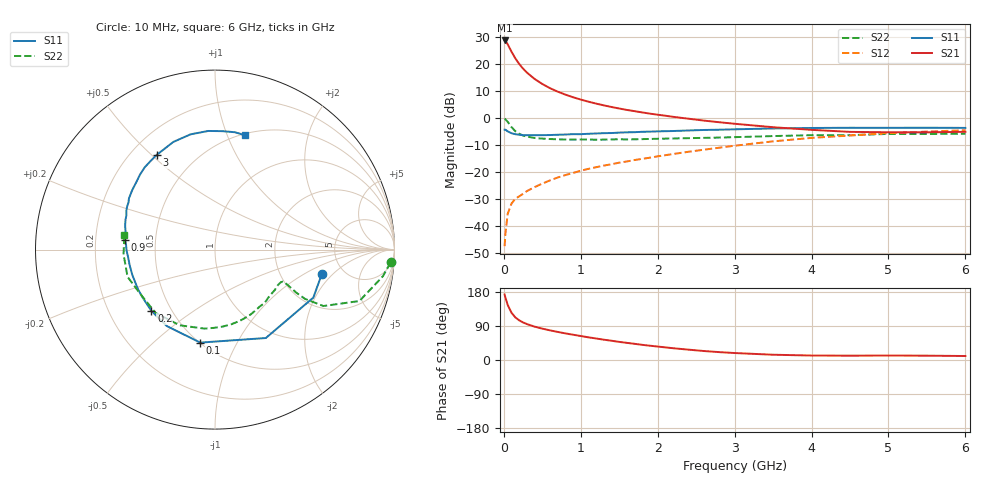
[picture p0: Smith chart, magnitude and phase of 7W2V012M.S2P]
! Infineon Technologies  Discrete & RF Semiconductors
! BFS17W
! Si NPN RF Bipolar Junction Transistor in SOT323
! VCE = 2 V  IC = 12 mA
! Common Emitter S-Parameters:  August  1999
# GHz  S  MA  R  50
!  f  S11  S21  S12  S22
! GHz  MAG  ANG  MAG  ANG  MAG  ANG  MAG  ANG
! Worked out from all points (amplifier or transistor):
!   36 points, 10 MHz to 6 GHz, reference 50 ohm
!   highest |S21| = 28.7 dB at 10 MHz (marker M1)
!   |S21| within 3 dB of that: start of sweep to 78.9 MHz
!   unconditionally stable (mu >= 1): 344.6 MHz to 2.89 GHz; 4.095 GHz to end of sweep
!   at 250 MHz: K = 0.88, MSG = 23.1 dB, |S12| = -28.0 dB
!   at 1.4 GHz: K = 1.24, MAG = 7.6 dB, |S12| = -17.0 dB
!   at 6 GHz: K = 1.09, MAG = -2.1 dB, |S12| = -4.5 dB
!   S11 on the Smith chart (normalised r, x): 10 MHz: 3.43, -1.50; 100 MHz: 0.50, -0.72; 200 MHz: 0.39, -0.35; 900 MHz: 0.33, +0.05; 3 GHz: 0.30, +0.52; 6 GHz: 0.51, +1.16
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0.01  0.6103 -13.0  27.17 172.8  0.0043 84.0  0.9805 -4.2
0.02  0.6098 -26.0  26.55 164.9  0.0072 81.8  0.9475 -9.0
0.05  0.5682 -60.1  23.09 145.4  0.017 67.1  0.8541 -19.6
0.1  0.5247 -99.0  16.84 124.6  0.0264 56.1  0.6808 -27.5
0.15  0.5036 -122.2  12.64 112.3  0.0324 52.8  0.5711 -28.7
0.2  0.4921 -136.0  9.99 104.7  0.0359 53.1  0.5126 -27.9
0.25  0.4837 -146.0  8.191 99.1  0.0398 53.9  0.4755 -26.8
0.3  0.4827 -152.9  6.924 94.8  0.0448 56.1  0.4549 -26.1
0.4  0.4819 -163.2  5.282 88.0  0.0531 58.9  0.4288 -25.3
0.5  0.4835 -169.9  4.264 82.8  0.0615 61.0  0.4178 -25.3
0.6  0.4858 -174.9  3.565 78.2  0.0706 62.7  0.4101 -26.2
0.7  0.4924 -179.2  3.083 74.1  0.0799 63.8  0.4056 -27.8
0.9  0.505 173.7  2.424 66.7  0.097 65.0  0.4 -31.7
1.1  0.5128 167.0  2.009 59.8  0.1154 65.3  0.4003 -36.6
1.3  0.5262 161.2  1.717 53.6  0.1324 65.8  0.3998 -42.3
1.6  0.5455 153.8  1.414 45.2  0.158 66.0  0.4032 -51.1
2.2  0.5767 139.7  1.056 31.1  0.2168 65.6  0.4203 -70.6
3  0.6196 121.5  0.785 18.4  0.3085 61.1  0.4441 -97.5
3.5  0.6432 111.2  0.678 13.9  0.3717 56.5  0.4651 -114.9
4.5  0.6621 93.2  0.556 11.4  0.4764 43.8  0.4838 -149.0
5.5  0.6632 80.4  0.545 11.4  0.5622 31.7  0.5102 -177.0
6  0.6588 75.5  0.557 10.5  0.5963 25.9  0.5118 170.7
